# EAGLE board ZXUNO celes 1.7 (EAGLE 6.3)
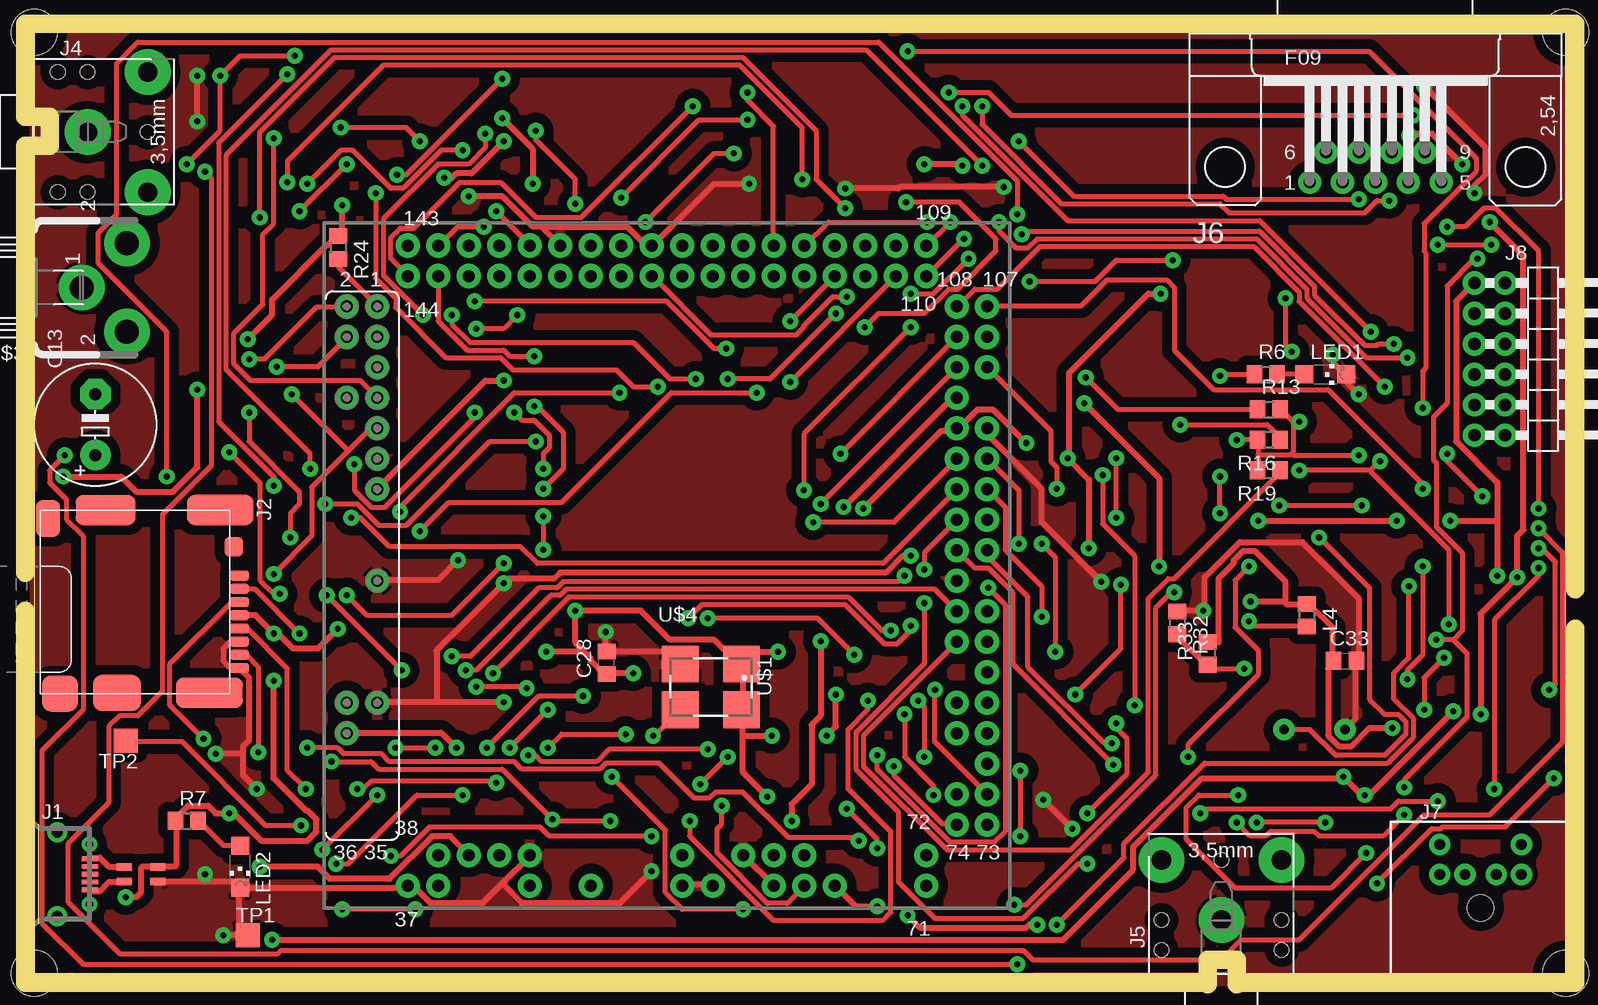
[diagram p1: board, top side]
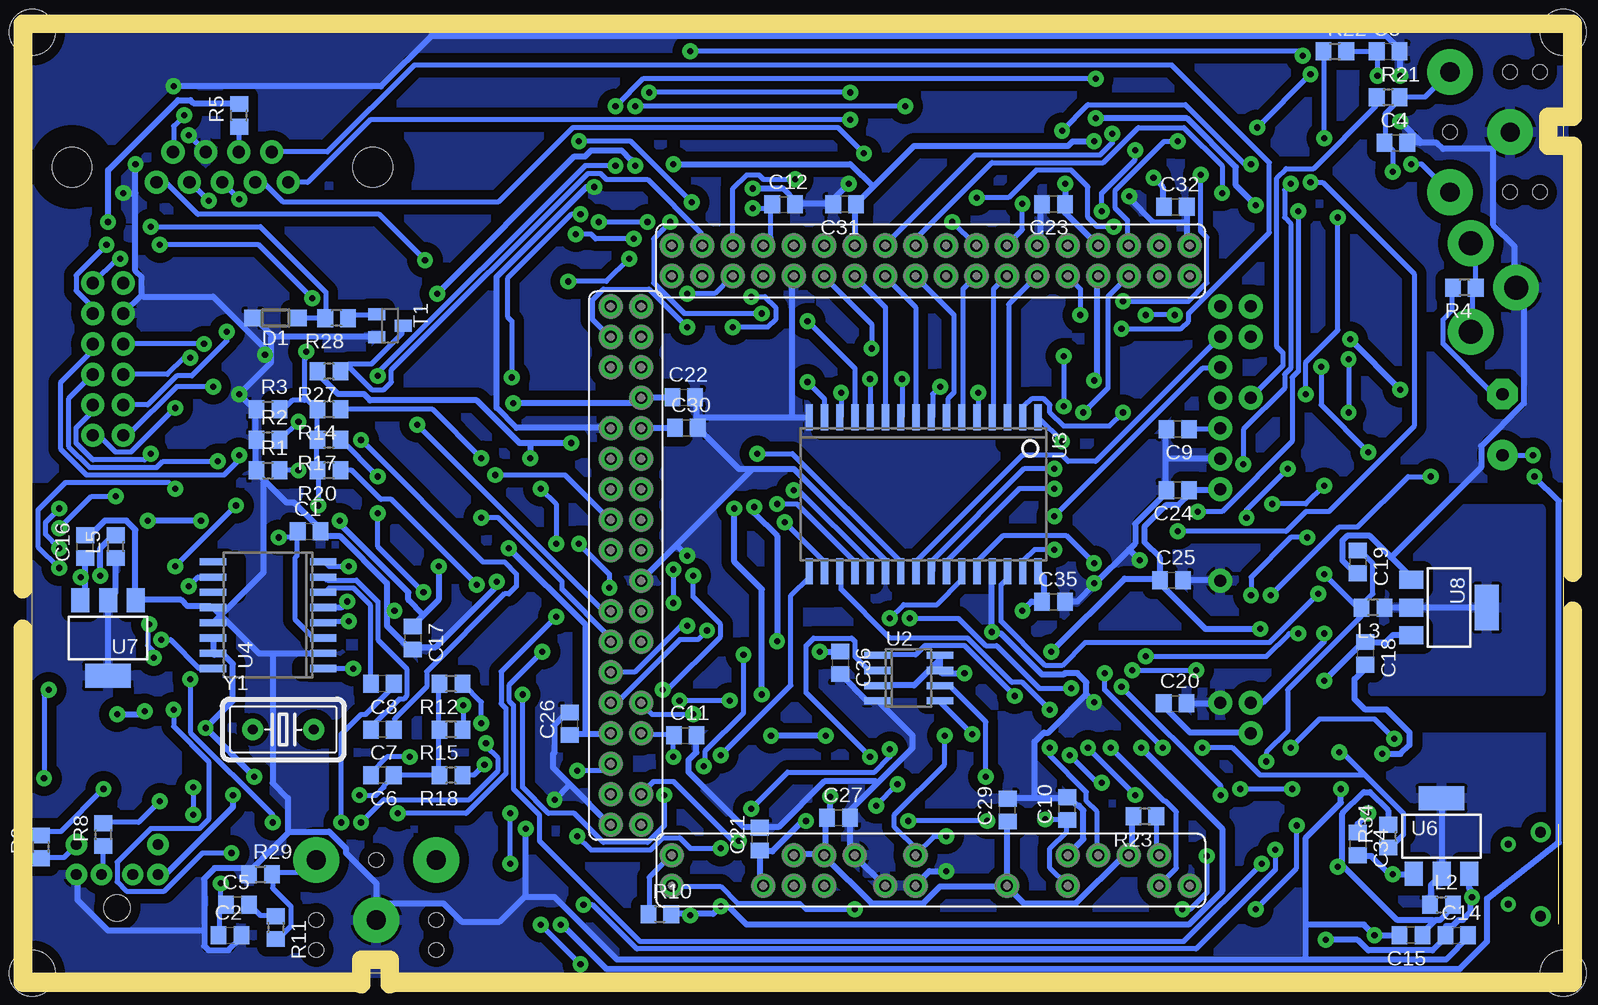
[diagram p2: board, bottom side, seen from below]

Size 127.61 x 78.41 mm. Coordinates in mm from the lower left corner, seen from the top.
Outline: 0,0 127.61,0 127.61,78.41 0,78.41 0,0
Copper layers (1*16): Top 0.035mm / dielectric 1.5mm / Bottom 0.035mm
Design rules "default *": minimum track width 16mil, minimum drill 20mil, track to track 8mil, track to pad 8mil, pad to pad 8mil, via to via 10mil, smd to smd 8mil, copper to edge 0mil, drill to drill 10mil, minimum pad ring 10mil, minimum via ring 16mil, stop-mask expansion 4mil, vias tented up to drill 0mil, thermal gap 10mil
Net classes: 0 default: width 0.381 mm, drill 0.203 mm, clearance 0.203 mm; 1 alimentacion: width 0.508 mm, drill 0.203 mm, clearance 0.203 mm
Holes 3.81 mm at 0,78.41 127.61,78.41 127.61,0 0,0
tRestrict: area 116.3,64.9 to 118.2,66.9; area 113.5,64.9 to 115.4,66.9; area 110.8,64.9 to 112.8,66.9; area 108,64.9 to 110,66.9; area 105.3,64.9 to 107.3,66.9; area 106.7,67.5 to 108.7,69.4; area 109.4,67.5 to 111.4,69.4; area 112.1,67.5 to 114,69.4; area 114.9,67.5 to 116.8,69.4; area 7.6,63.4 to 11.2,66.9; area 2.5,68.3 to 6.1,71.9; area 7.6,73.3 to 11.2,76.8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
bRestrict: area 108.7,19.8 to 109.7,20.8; area 103.6,19.8 to 104.7,20.9; area 61,31.3 to 63.4,32.2; area 43.6,31.6 to 46.6,32.3; area 43.6,44.1 to 46.5,45; area 110.6,31.6 to 111.3,34.4; area 113.8,33.9 to 114.7,34.5; area 104.5,25.1 to 105.2,25.7; area 104.5,29.6 to 105.4,34.5
vRestrict: area 50.8,21.4 to 58.4,27.8; area 102.2,24.1 to 113.7,35.6; area 92.7,-2.5 to 104.8,11.4; area 119.4,43.6 to 127,58.8; area -1.3,3.8 to 5.7,12.7; area 7,7.6 to 13.3,15.9; area 112.9,-0.3 to 128.1,12.4; area 96.3,64.3 to 102.6,78.9; area 121.3,64.3 to 127,78.9; area 99.6,74.7 to 124.3,78.5; area -2,64.4 to 11.9,76.5; area 0.6,20.3 to 18.4,40.6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
Milling: 15 lines

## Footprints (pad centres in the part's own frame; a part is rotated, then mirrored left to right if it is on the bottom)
C0805 = smd 1.3 x 1.5: 1 -0.95,0; 2 0.95,0
E5-10,5 = drill 1.016 pad 2.54: + -2.54,0 | drill 1.016 pad 2.54 octagon: - 2.54,0
SOD123 = smd 1.4 x 1.4: A 1.9,0; C -1.9,0
MICRO_USB = smd 1.35 x 0.4: 1 2.73,1.3; 2 2.73,0.65; 3 2.73,0; 4 2.73,-0.65; 5 2.73,-1.3 | drill 0.6 pad 1.27: P$1 2.7,2.5; P$2 2.7,-2.5 | drill 0.9 pad 1.676: P$3 0,3.5; P$4 0,-3.5
MICRO_SD_CONNECTOR = smd 0.8 x 1.6: 1 -2.03,8.2; 2 -0.93,8.2; 3 0.17,8.2; 4 1.27,8.2; 5 2.37,8.2; 6 3.47,8.2; 7 4.57,8.2; 8 5.67,8.2 | smd 2.54 x 5.588: 9 7.735,5.7; 14 -7.49,6.6 | smd 3 x 4: 10 7.735,-2 | smd 3 x 3: 11 7.81,-6.75 | smd 3 x 2: 12 -6.79,-7.75 | smd 2.5 x 5: 13 -7.49,-2.95 | smd 1.6 x 1.55: 15 -4.43,7.725
STX = drill 1.6 pad 3.81: P$1 -0.762,-0.127; P$2 4.242,-5.131; P$3 4.242,4.877 | hole 1.2: -3.251,4.877; -0.762,4.877; -0.762,-5.131; -3.251,-5.131; 4.242,-0.127
F09H = drill 1.016 pad 1.93: 1 -5.486,-1.27; 2 -2.743,-1.27; 3 0,-1.27; 4 2.743,-1.27; 5 5.486,-1.27; 6 -4.115,1.27; 7 -1.372,1.27; 8 1.372,1.27; 9 4.115,1.27 | hole 3.302: -12.522,0; 12.522,0
MDIN06SS = drill 0.9 pad 1.778: 1 1.3,8.5; 2 -1.3,8.5; 3 3.4,8.5; 4 -3.4,8.5; 5 3.4,11; 6 -3.4,11 | hole 2.2: 0,5.716
2X06/90 = drill 1.016 pad 1.93: 1 -6.35,-6.35; 2 -6.35,-3.81; 3 -3.81,-6.35; 4 -3.81,-3.81; 5 -1.27,-6.35; 6 -1.27,-3.81; 7 1.27,-6.35; 8 1.27,-3.81; 9 3.81,-6.35; 10 3.81,-3.81; 11 6.35,-6.35; 12 6.35,-3.81
CHOKE_COMM = smd 1.27 x 0.635: P$1 -1.4,0.6; P$2 -1.4,-0.6; P$3 1.4,-0.6; P$4 1.4,0.6
0805 = smd 1.3 x 1.5: 1 -0.95,0; 2 0.95,0
CHIPLED_1206 = smd 1.5 x 1.5: A 0,-1.75; C 0,1.75
R0805 = smd 1.3 x 1.5: 1 -0.95,0; 2 0.95,0
SOT23 = smd 1 x 1.4: 1 -0.95,-1.1; 2 0.95,-1.1; 3 0,1.1
TP20SQ = smd 2 x 2: TP 0,0
SO-08 = smd 0.6 x 2.2: 1 -1.905,-2.6; 2 -0.635,-2.6; 3 0.635,-2.6; 4 1.905,-2.6; 5 1.905,2.6; 6 0.635,2.6; 7 -0.635,2.6; 8 -1.905,2.6
SOIC32 = smd 0.6 x 2.2: 1 -9.525,-6.416; 2 -8.255,-6.416; 3 -6.985,-6.416; 4 -5.715,-6.416; 5 -4.445,-6.416; 6 -3.175,-6.416; 7 -1.905,-6.416; 8 -0.635,-6.416; 9 0.635,-6.416; 10 1.905,-6.416; 11 3.175,-6.416; 12 4.445,-6.416; 13 5.715,-6.416; 14 6.985,-6.416; 15 8.255,-6.416; 16 9.525,-6.416; 17 9.525,6.416; 18 8.255,6.416; 19 6.985,6.416; 20 5.715,6.416; 21 4.445,6.416; 22 3.175,6.416; 23 1.905,6.416; 24 0.635,6.416; 25 -0.635,6.416; 26 -1.905,6.416; 27 -3.175,6.416; 28 -4.445,6.416; 29 -5.715,6.416; 30 -6.985,6.416; 31 -8.255,6.416; 32 -9.525,6.416
SO16W = smd 0.6 x 2.2: 1 -4.445,-4.6; 2 -3.175,-4.6; 3 -1.905,-4.6; 4 -0.635,-4.6; 5 0.635,-4.6; 6 1.905,-4.6; 7 3.175,-4.6; 8 4.445,-4.6; 9 4.445,4.6; 10 3.175,4.6; 11 1.905,4.6; 12 0.635,4.6; 13 -0.635,4.6; 14 -1.905,4.6; 15 -3.175,4.6; 16 -4.445,4.6
SOT223 = smd 1.5 x 2: 1 -2.3,-3.15; 2 0,-3.15; 3 2.3,-3.15 | smd 3.8 x 2: 4 0,3.15
SM77H = smd 3.048 x 3.048: 1 -2.55,-1.9; 2 2.55,-1.9; 3 2.55,1.9; 4 -2.55,1.9
RCA_PACK = drill 2 pad 3.81: 1 0,-3.945; 2 3.688,-7.72; 2@1 -3.688,-7.72
TQ144_DIP_INCOMPLETO_2CARAS = drill 1 pad 2.007: P1 -24.13,21.59; P2 -26.67,21.59; P3 -24.13,19.05; P4 -26.67,19.05; P5 -24.13,16.51; P7 -24.13,13.97; P8 -26.67,13.97; P9 -24.13,11.43; P11 -24.13,8.89; P13 -24.13,6.35; P19 -24.13,-1.27; P27 -24.13,-11.43; P28 -26.67,-11.43; P30 -26.67,-13.97; P37 -21.59,-26.67; P39 -19.05,-26.67; P40 -19.05,-24.13; P42 -16.51,-24.13; P44 -13.97,-24.13; P45 -11.43,-26.67; P46 -11.43,-24.13; P49 -6.35,-26.67; P55 1.27,-26.67; P56 1.27,-24.13; P57 3.81,-26.67; P60 6.35,-24.13; P61 8.89,-26.67; P62 8.89,-24.13; P63 11.43,-26.67; P64 11.43,-24.13; P65 13.97,-26.67; P71 21.59,-26.67; P72 21.59,-24.13; P73 26.67,-21.59; P74 24.13,-21.59; P75 26.67,-19.05; P76 24.13,-19.05; P77 26.67,-16.51; P79 26.67,-13.97; P80 24.13,-13.97; P81 26.67,-11.43; P82 24.13,-11.43; P83 26.67,-8.89; P85 26.67,-6.35; P86 24.13,-6.35; P87 26.67,-3.81; P88 24.13,-3.81; P90 24.13,-1.27; P91 26.67,1.27; P92 24.13,1.27; P93 26.67,3.81; P94 24.13,3.81; P95 26.67,6.35; P96 24.13,6.35; P97 26.67,8.89; P98 24.13,8.89; P99 26.67,11.43; P100 24.13,11.43; P102 24.13,13.97; P103 26.67,16.51; P104 24.13,16.51; P105 26.67,19.05; P106 24.13,19.05; P107 26.67,21.59; P108 24.13,21.59; P109 21.59,26.67; P110 21.59,24.13; P111 19.05,26.67; P112 19.05,24.13; P113 16.51,26.67; P114 16.51,24.13; P115 13.97,26.67; P116 13.97,24.13; P117 11.43,26.67; P118 11.43,24.13; P119 8.89,26.67; P120 8.89,24.13; P121 6.35,26.67; P122 6.35,24.13; P123 3.81,26.67; P124 3.81,24.13; P125 1.27,26.67; P126 1.27,24.13; P127 -1.27,26.67; P128 -1.27,24.13; P129 -3.81,26.67; P130 -3.81,24.13; P131 -6.35,26.67; P132 -6.35,24.13; P133 -8.89,26.67; P134 -8.89,24.13; P135 -11.43,26.67; P136 -11.43,24.13; P137 -13.97,26.67; P138 -13.97,24.13; P139 -16.51,26.67; P140 -16.51,24.13; P141 -19.05,26.67; P142 -19.05,24.13; P143 -21.59,26.67; P144 -21.59,24.13
HC18U-V = drill 0.813 pad 1.778: 1 -2.54,0; 2 2.54,0

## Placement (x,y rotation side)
C1  15pF  [C0805]  104.52,36.83 0 bottom
C2  10nF  [C0805]  111.12,3.17 0 bottom
C3  10nF  [C0805]  14.61,76.83 0 bottom
C4  10nF  [C0805]  13.97,69.22 0 bottom
C5  100nF  [C0805]  110.49,5.71 0 bottom
C6  100nF  [C0805]  98.42,16.51 180 bottom
C7  100nF  [C0805]  98.42,20.32 180 bottom
C8  100nF  [C0805]  98.42,24.13 180 bottom
C9  100nF  [C0805]  32.14,45.35 180 bottom
C10  100nF  [C0805]  41.34,13.73 90 bottom
C11  100nF  [C0805]  73.18,19.82 0 bottom
C12  100nF  [C0805]  64.98,64.07 0 bottom
C13  220uF  [E5-10,5]  5.08,45.72 90 top
C14  4,7uF  [C0805]  8.89,3.17 0 bottom
C15  4,7uF  [C0805]  12.7,3.17 180 bottom
C16  4,7uF  [C0805]  123.19,35.56 90 bottom
C17  4,7uF  [C0805]  95.89,27.94 270 bottom
C18  4,7uF  [C0805]  16.51,26.67 270 bottom
C19  4,7uF  [C0805]  17.14,34.29 270 bottom
C20  100nF  [C0805]  32.36,22.49 0 bottom
C21  100nF  [C0805]  66.96,11.19 90 bottom
C22  100nF  [C0805]  73.31,48.02 0 bottom
C23  100nF  [C0805]  42.5,64.09 180 bottom
C24  100nF  [C0805]  32.14,40.27 180 bottom
C25  100nF  [C0805]  32.67,32.78 0 bottom
C26  100nF  [C0805]  82.79,20.8 90 bottom
C27  100nF  [C0805]  60.41,12.98 0 bottom
C28  100nF  [C0805]  47.69,25.88 90 top
C29  100nF  [C0805]  46.33,13.6 90 bottom
C30  100nF  [C0805]  73.09,45.48 0 bottom
C31  100nF  [C0805]  59.9,64.09 180 bottom
C32  100nF  [C0805]  32.34,63.87 0 bottom
C33  100nF  [C0805]  109.22,26.04 0 top
C34  4,7uF  [C0805]  17.14,10.79 270 bottom
C35  100nF  [C0805]  42.5,30.96 0 bottom
C36  100nF  [C0805]  60.28,25.88 270 bottom
D1  [SOD123]  107.31,54.61 180 bottom
J1  CON_MICRO_USB  [MICRO_USB]  1.91,8.26 0 top
J2  MICROSD_SPI_MODE  [MICRO_SD_CONNECTOR]  8.89,31.11 270 top
J4  JACK_STEREO  [STX]  5.21,70.23 0 top
J5  JACK_STEREO  [STX]  98.81,5.21 90 top
J6  [F09H]  111.76,67.18 0 top
J7  [MDIN06SS]  120.52,-0.25 0 top
J8  JTAG_RGB  [2X06/90]  126.36,51.18 270 top
L1  BOBINA_VCC_ZXUNO  [CHOKE_COMM]  8.89,8.26 0 top
L2  FERRITE  [0805]  10.16,5.71 0 bottom
L3  FERRITE  [0805]  15.88,30.48 180 bottom
L4  FERRITE  [0805]  106.05,29.84 270 top
L5  FERRITE  [0805]  120.65,35.56 90 bottom
LED1  [CHIPLED_1206]  107.57,49.91 270 top
LED2  [CHIPLED_1206]  17.14,8.89 180 top
R1  75  [R0805]  107.95,41.91 0 bottom
R2  75  [R0805]  107.95,44.45 0 bottom
R3  75  [R0805]  107.95,46.99 0 bottom
R4  75  [R0805]  8.26,57.15 180 bottom
R5  270  [R0805]  110.36,71.5 90 bottom
R6  220  [R0805]  102.62,49.91 0 top
R7  220  [R0805]  12.7,12.7 0 top
R8  270  [R0805]  121.67,11.56 90 bottom
R9  270  [R0805]  126.87,10.54 90 bottom
R10  330  [R0805]  75.3,4.94 0 bottom
R11  470  [R0805]  107.31,3.81 270 bottom
R12  470  [R0805]  92.71,24.13 180 bottom
R13  470  [R0805]  102.87,46.99 0 top
R14  470  [R0805]  102.87,46.99 180 bottom
R15  1K  [R0805]  92.71,20.32 180 bottom
R16  1K  [R0805]  102.87,44.45 180 top
R17  1K  [R0805]  102.87,44.45 180 bottom
R18  2K  [R0805]  92.71,16.51 180 bottom
R19  2K  [R0805]  102.87,41.91 180 top
R20  2K  [R0805]  102.87,41.91 180 bottom
R21  3K9  [R0805]  14.61,73.03 0 bottom
R22  3K9  [R0805]  19.05,76.83 0 bottom
R23  4K7  [R0805]  34.88,13.07 180 bottom
R24  4K7  [R0805]  25.32,60.48 270 top
R27  1OK  [R0805]  102.87,50.16 180 bottom
R28  10K  [R0805]  102.23,54.61 180 bottom
R29  10K  [R0805]  108.58,8.26 0 bottom
R32  0  [R0805]  95.25,29.21 270 top
R33  0  [R0805]  97.79,26.67 90 top
R34  10K  [R0805]  14.61,11.43 90 bottom
T1  BC846  [SOT23]  97.79,53.98 270 bottom
TP1  TPTP20SQ  [TP20SQ]  17.78,3.17 0 top
TP2  TPTP20SQ  [TP20SQ]  7.64,19.38 180 top
U2  W25X40BV  [SO-08]  54.56,24.61 270 bottom
U3  CY62148EV30  [SOIC32]  53.32,39.93 180 bottom
U4  AD724JR  [SO16W]  107.95,29.84 90 bottom
U6  LD117AS33TR  [SOT223]  10.16,11.43 0 bottom
U7  LD117AS25TR  [SOT223]  121.28,27.94 180 bottom
U8  LD117AS12TR  [SOT223]  9.53,30.48 270 bottom
U$1  SIT1602AC-83  [SM77H]  56.38,23.87 180 top
U$3  RCA_VIDEO  [RCA_PACK]  0,57.15 90 top
U$4  [TQ144_DIP_INCOMPLETO_2CARAS]  52.72,33.98 0 top
Y1  4.43M/3.58M  [HC18U-V]  106.68,20.32 0 bottom

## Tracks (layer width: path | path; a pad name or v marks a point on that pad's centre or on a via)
1.2V  (via drill 0.51)
  Top 0.406: v24.77,17.65 28.07,17.65 28.7,17.02 38.99,17.02 v43.18,12.83 43.31,12.7 v48.01,12.7 | v19.94,33.27 23.11,36.45 23.11,40.51 26.16,43.56 | 26.16,43.56 27.94,45.34 28.57,45.34 U$4.P9 | v67.56,63.75 65.15,66.17 65.15,70.23 59.05,76.33 25.02,76.33 18.8,70.1 v18.8,62.99 | 26.16,43.56 v21.46,48.26 | v74.17,18.03 74.17,22.23 v73.66,22.73 | v69.47,22.73 69.47,21.97 67.82,20.32 67.82,15.37 71.37,11.81 71.37,5.08 70.74,4.45 61.59,4.45 54.61,11.43 v54.61,12.7
  Bottom 0.406: C9.1 31.11,45.34 28.7,45.34 U$4.P9 | U$4.P45 41.4,7.37 42.8,8.76 42.8,10.41 41.4,11.81 41.4,12.7 C10.1 41.53,12.83 v43.18,12.83 | v24.77,17.65 24.77,18.41 22.99,20.19 22.99,23.62 16.89,29.72 16.89,30.35 L3.2 | U$4.P115 66.67,60.71 66.04,61.34 66.04,64.01 C12.1 66.17,63.75 v67.56,63.75 | C19.1 17.14,35.18 16.89,35.18 15.88,34.16 15.88,31.62 16.89,30.61 L3.2 | v19.94,33.27 17.4,30.73 17.02,30.73 L3.2 | v18.8,62.99 18.8,53.59 21.46,50.93 v21.46,48.26 | U$4.P80 76.83,19.94 74.17,19.94 C11.1 74.17,19.68 v74.17,18.03 | v69.47,22.73 v73.66,22.73 | v48.01,12.7 v54.61,12.7
2.5V  (via drill 0.51)
  Top 0.508: v63.12,12.7 63.12,14.1 64.77,15.75 64.77,20.7 65.53,21.46 v65.53,27.69 | v67.44,38.86 76.45,47.88 76.83,47.88 U$4.P102 | v41.53,65.79 41.53,68.71 v38.99,71.25 | v25.65,64.01 25.65,61.85 25.4,61.59 R24.1 25.15,61.34 24.51,60.71 24.38,60.71 19.81,56.13 19.81,54.86 v17.78,52.83 | v70.23,5.59 68.45,5.59 66.8,7.24 U$4.P65 | v35.18,18.8 33.91,20.07 26.16,20.07 U$4.P30 | 121.92,37.72 121.92,40.89 118.49,44.32 118.49,56.01 J8.1 | 121.92,37.72 v121.92,33.15 | v93.73,33.91 93.73,41.27 v87.5,47.5 | v13.59,48.64 13.59,42.16 11.56,40.13 8.51,40.13 7.24,41.4 v2.41,41.4 | v83.57,4.06 82.93,4.06 82.68,3.81 73.79,3.81 v72.77,4.83 | v117.98,37.72 121.92,37.72 | v101.98,37.72 v113.54,37.72
  Bottom 0.508: C22.1 74.3,48.01 76.83,48.01 U$4.P102 77.09,47.88 77.47,47.5 v87.5,47.5 | U$4.P137 38.86,60.71 41.53,63.37 41.53,64.01 C23.1 41.53,64.26 v41.53,65.79 | U$4.P65 66.8,7.37 66.93,7.49 66.93,10.16 C21.1 66.67,10.16 65.91,10.16 63.37,12.7 v63.12,12.7 | C20.1 33.27,22.48 33.27,22.23 31.11,20.07 26.16,20.07 U$4.P30 | v65.53,27.69 65.53,36.45 67.44,38.35 v67.44,38.86 | v38.99,71.25 31.37,71.25 27.3,67.18 27.3,65.66 v25.65,64.01 | 72.77,4.95 70.87,4.95 v70.23,5.59 70.1,5.46 69.47,5.46 68.07,4.06 31.24,4.06 28.45,6.86 28.45,12.06 v35.18,18.8 | 72.77,4.95 74.3,4.95 R10.2 | v121.92,33.15 121.92,35.43 120.9,36.45 120.65,36.45 L5.2 | 95,29.84 93.73,31.11 v93.73,33.91 | 95,29.84 95.89,28.96 C17.1 | v13.59,48.64 v17.78,52.83 | v2.41,41.4 0.38,39.37 0.38,10.92 6.35,6.22 6.35,2.67 8.64,0.38 79.76,0.38 83.44,4.06 v83.57,4.06 | v72.77,4.83 72.77,4.95 | v113.54,37.72 v117.98,37.72 | v101.98,37.72 101.98,37.47 96.27,31.75 96.27,31.11 95,29.84
3.3V  (via drill 0.51)
  Top 0.508: v49.91,25.02 47.75,25.02 C28.1 47.5,24.89 46.35,26.04 46.35,26.29 45.72,26.92 | 45.72,26.92 45.09,27.56 v45.09,30.23 50.55,30.23 52.96,27.81 56.64,27.81 58.67,25.78 U$1.1 | U$1.1 59.05,25.53 59.05,21.97 U$1.4 59.05,21.72 59.05,19.81 | 59.05,19.81 59.05,16.76 v61.09,14.73 | v42.67,26.8 45.59,26.8 45.72,26.92 | J2.4 18.41,29.84 v19.94,28.32 20.07,28.19 20.45,28.19 21.59,27.05 23.62,27.05 v25.27,28.7 | v61.98,26.8 57.91,26.8 U$1.1 | v69.09,38.73 75.56,45.21 76.71,45.21 U$4.P100 77.09,45.47 78.61,46.99 79.88,46.99 v82.68,44.2 | v66.8,23.24 66.8,20.57 v66.04,19.81 | 59.05,19.81 v61.47,19.81 | v39.12,49.4 37.59,49.4 28.57,40.39 U$4.P13 | v18.8,8.89 23.62,8.89 24.64,7.87 29.59,7.87 33.15,11.43 34.67,11.43 36.2,9.91 U$4.P42 | v34.16,66.29 34.8,66.29 35.18,66.67 36.45,66.67 v39.12,69.34 | v87.88,35.43 87.88,41.15 v86.11,42.93 86.23,43.05 86.23,50.04 92.84,56.64 v93.85,56.64 | v74.17,67.44 77.22,67.44 v77.34,67.31
  Bottom 0.508: U$4.P13 28.7,40.26 31.11,40.26 C24.1 31.11,40.01 32.13,38.99 33.15,38.99 34.92,37.21 34.92,35.94 33.66,34.67 33.66,32.89 C25.1 | C30.1 74.04,45.47 76.83,45.47 U$4.P100 | U$4.P121 59.05,60.71 59.05,63.88 C31.1 58.8,64.26 57.53,65.53 | U3.32 43.69,33.4 43.31,33.02 43.31,31.37 43.43,31.24 43.43,30.99 C35.1 43.69,30.99 44.32,30.99 v45.09,30.23 | v49.91,25.02 51.82,25.02 51.94,25.15 U2.7 51.94,25.4 51.94,26.04 | 51.94,26.04 51.94,26.42 U2.8 | U2.3 57.15,24 54.1,24 52.07,26.04 51.94,26.04 | R23.2 35.94,12.95 35.94,10.16 36.2,9.91 U$4.P42 36.45,9.78 36.7,9.78 40.64,5.84 44.96,5.84 46.23,7.11 U$4.P49 | C29.1 46.35,12.57 46.35,7.37 U$4.P49 | U$4.P62 61.59,9.91 61.47,10.03 61.47,12.95 C27.1 61.34,13.21 61.09,13.46 v61.09,14.73 | U$4.P49 46.61,7.24 51.94,7.24 53.34,5.84 57.66,5.84 61.47,9.65 U$4.P62 | U$4.P64 64.14,9.91 61.85,9.91 U$4.P62 | v42.67,26.8 36.58,32.89 33.91,32.89 C25.1 | v19.94,28.32 19.94,27.69 25.02,22.61 26.04,22.61 U$4.P28 | v61.98,26.8 60.33,26.8 C36.1 | v69.09,38.73 69.09,34.29 66.8,32 v66.8,23.24 | v61.47,19.81 v66.04,19.81 | 10.79,4.32 10.67,4.45 10.29,4.45 9.27,5.46 9.27,5.71 L2.2 | 10.79,4.32 11.68,3.43 11.68,3.17 C15.1 | R34.2 14.61,13.59 16.13,15.11 16.64,15.11 18.41,13.34 18.41,9.02 | 18.41,9.02 13.84,4.45 10.92,4.45 10.79,4.32 | v39.12,49.4 38.86,49.66 38.86,58.04 U$4.P138 | v18.8,8.89 18.54,8.89 18.41,9.02 | v25.27,28.7 29.84,28.7 33.66,32.51 C25.1 | v34.16,66.29 33.4,65.53 33.4,63.88 C32.1 | v39.12,69.34 40.89,69.34 41.27,68.96 54.1,68.96 57.53,65.53 | 81.53,19.94 79.5,19.94 U$4.P79 | 81.53,19.94 82.68,19.94 C26.1 | v82.68,44.2 86.11,44.2 | 86.11,44.2 87,44.2 90.55,47.75 99.44,47.75 99.95,48.26 102.11,48.26 103.76,49.91 103.76,50.16 R27.2
  Bottom 0.508: 81.53,19.94 81.53,29.08 v87.88,35.43 | 86.11,44.2 v86.11,42.93 | 57.53,65.53 59.44,67.44 v74.17,67.44 | v77.34,67.31 77.72,67.69 77.72,67.82 78.49,68.58 81.03,68.58 81.53,68.07 82.42,68.07 v93.85,56.64
5V  (via drill 0.51)
  Top 0.508: v7.62,6.35 8.51,6.35 8.89,6.73 8.89,8.76 9.02,8.89 10.03,8.89 L1.P$4 10.41,8.89 11.68,8.89 11.81,9.02 11.81,12.7 R7.1 11.68,12.83 12.83,13.97 14.48,13.97 15.11,13.34 v16.26,13.34 16.38,13.21 16.76,13.21 18.92,11.05 22.73,11.05 23.5,11.81 23.5,12.83 22.73,13.59 22.61,13.59 19.94,16.26 v19.94,24.38 | 104.27,30.99 104.27,30.86 104.39,30.73 106.05,30.73 L4.1 106.17,30.61 106.43,30.61 108.2,28.83 108.2,26.29 C33.1 108.2,25.78 107.82,25.4 107.82,19.81 108.71,18.92 109.73,18.92 111.25,20.45 v113.16,20.45 | 104.27,30.99 104.27,32.64 101.73,35.18 100.71,35.18 99.95,34.42 99.95,34.16 98.68,32.89 98.68,27.56 97.79,27.56 R33.2 | 104.27,30.99 v101.35,30.99 | v121.28,62.61 124.08,59.82 124.08,36.96 123.57,36.45 v123.57,33.02 120.52,29.97 v120.52,21.59 | v118.24,21.84 111.38,14.99 111,14.99 v110.87,14.86 110.62,14.86 v109.09,16.38 108.97,16.26 97.28,16.26 91.57,10.54 91.57,8.64 85.72,2.79 v19.81,2.79
  Bottom 0.508: 7.75,6.35 7.75,6.99 7.87,7.11 7.87,8.26 U6.3 | 7.75,6.35 7.75,5.08 8.38,4.45 8.76,4.45 9.27,3.94 9.78,3.94 9.78,3.17 C14.1 9.78,3.05 10.92,1.91 16.26,1.91 17.14,2.79 v19.81,2.79 | 14.86,27.56 16.51,27.56 C18.1 16.64,27.43 16.89,27.43 v19.94,24.38 | 14.86,27.56 14.22,28.19 12.7,28.19 U8.3 | 14.73,27.43 14.86,27.56 | v7.62,6.35 7.75,6.35 | U4.5 101.85,30.48 v101.35,30.99 | 123.19,33.02 123.19,31.5 123.57,31.11 U7.3 | 123.19,33.02 C16.1 | v121.28,62.61 121.28,66.93 115.44,72.77 114.43,72.77 114.17,72.52 110.36,72.52 R5.2 | 123.19,33.02 v123.57,33.02 | C34.1 17.14,12.45 v16.26,13.34 | U4.14 112.52,27.94 112.52,26.67 U4.15 112.39,26.54 111.63,26.54 110.87,25.78 110.87,22.73 v113.16,20.45 v109.09,16.38 | v110.87,14.86 110.87,13.84 116.46,8.26 117.09,8.26 J7.4 | v118.24,21.84 118.49,21.59 v120.52,21.59
B  (via drill 0.51)
  Top 0.406: 111.38,41.91 v105.41,41.91 | v112.14,42.67 111.38,41.91 | v100.33,14.86 97.03,14.86 96.01,13.84 96.01,11.18 100.08,7.11 108.08,7.11 v111,10.03 | v115.82,21.97 115.82,24.64 v117.47,26.29 | v117.86,29.08 117.86,35.31 111.38,41.78 111.38,41.91
  Bottom 0.406: R12.2 93.73,24.13 93.73,20.45 R15.2 93.73,20.19 93.73,16.64 R18.2 C6.1 97.54,16.38 98.3,15.62 98.3,15.49 98.93,14.86 v100.33,14.86 | v105.41,41.91 R1.2 | v112.14,42.67 116.71,42.67 117.22,42.16 122.81,42.16 124.59,43.94 124.59,47.88 J8.8 | v111,10.03 113.41,10.03 116.59,6.86 119.76,6.86 120.52,7.62 120.52,9.27 117.73,12.06 113.67,12.06 112.9,12.83 112.9,17.65 115.82,20.57 v115.82,21.97 | v117.47,26.29 117.35,26.42 117.35,26.67 117.98,27.3 117.98,28.96 v117.86,29.08
B0  (via drill 0.51)
  Top 0.406: v89.92,17.4 81.53,25.78 81.53,31.75 79.5,33.78 78.36,33.78 76.96,35.18 U$4.P92
  Bottom 0.406: R18.1 90.81,16.51 v89.92,17.4
B1  (via drill 0.51)
  Top 0.406: v91.69,22.35 91.69,34.8 89.03,37.47 v89.03,41.53
  Bottom 0.406: v91.69,22.35 91.69,20.32 R15.1 | v89.03,41.53 83.19,41.53 79.5,37.85 U$4.P93
B2  (via drill 0.51)
  Top 0.406: v90.17,20.83 90.17,20.45 91.06,19.56 91.06,16.64 v87.76,13.34 | v87.76,9.14 87,9.14 82.42,4.57 75.06,4.57 72.01,7.62 72.01,13.46 68.45,17.02 68.45,20.07 74.17,25.78 v74.17,30.86 | v74.17,33.66 74.17,35.05 76.83,37.72 U$4.P94
  Bottom 0.406: v90.17,20.83 90.17,22.61 91.69,24.13 R12.1 | v87.76,9.14 v87.76,13.34 | v74.17,33.66 v74.17,30.86
CLK  (via drill 0.51)
  Top 0.406: v22.23,12.32 19.3,12.32 12.32,19.3 7.75,19.3 TP2.TP | v31.75,5.33 v25.65,5.33 | v29.72,9.78 30.48,9.78 32.89,12.19 42.16,12.19 42.93,11.43 v51.44,11.43 | v51.56,19.81 51.69,19.81 53.72,21.84 U$1.3
  Bottom 0.406: v22.23,12.32 22.23,8.76 v25.65,5.33 | v31.75,5.33 31.11,5.33 29.72,6.73 v29.72,9.78 | v51.44,11.43 52.45,11.43 53.98,9.91 U$4.P56 53.85,10.29 55.75,12.19 55.75,13.21 51.56,17.4 v51.56,19.81
CSYNC  (via drill 0.51)
  Top 0.406: 118.24,27.81 v116.84,27.81 | 118.24,27.81 119,28.57 119,35.05 116.84,37.21 116.84,42.55 116.59,42.8 116.59,46.35 117.73,47.5 117.73,57.28 120.02,59.56 v120.27,59.56 | v89.79,19.18 89.15,19.18 82.8,25.53 82.8,31.37 79.5,34.67 79.5,35.18 U$4.P91 | v100.2,12.57 101.35,11.43 102.62,11.43 103,11.81 106.68,11.81 107.06,11.43 112.39,11.43 v114.17,13.21 | v114.17,15.49 114.17,16.13 119.38,21.34 119.38,26.67 118.24,27.81
  Bottom 0.406: U4.16 113.67,25.4 116.08,27.81 v116.84,27.81 | v120.27,59.56 120.52,59.56 J8.2 | v89.79,19.18 89.79,18.92 88.77,17.91 88.77,16.89 91.19,14.48 98.3,14.48 v100.2,12.57 | v114.17,15.49 v114.17,13.21
EAR
  Bottom 0.406: 101.35,50.67 101.85,50.16 R27.1 | 101.35,50.67 101.22,50.8 99.31,50.8 96.77,53.34 96.77,53.98 T1.3 | 101.35,50.67 99.31,48.64 98.3,48.64 97.66,49.28 97.66,50.29 81.28,66.67 80.26,66.67 79.76,66.17 76.33,66.17 71.88,61.72 71.88,60.71 U$4.P111
FLASH_CS  (via drill 0.51)
  Top 0.406: v45.72,23.11 42.04,23.11 v37.72,18.8
  Bottom 0.406: v45.72,23.11 49.91,27.3 53.21,27.3 53.98,26.54 57.15,26.54 U2.1 | v37.72,18.8 33.27,14.35 33.15,14.35 32.26,13.46 32.26,8.76 33.66,7.37 U$4.P39
FLASH_MISO  (via drill 0.51)
  Top 0.406: v55.5,15.75 v57.78,18.03 | v57.28,13.97 57.28,12.45 56.9,12.06 56.9,10.03 61.09,5.84 62.74,5.84 64.14,7.24 U$4.P63
  Bottom 0.406: v57.78,18.03 63.12,23.37 63.12,27.3 62.48,27.94 59.31,27.94 59.05,27.69 59.05,26.42 57.91,25.27 57.28,25.27 U2.2 | v57.28,13.97 v55.5,15.75
FLASH_MOSI  (via drill 0.51)
  Top 0.406: v49.28,19.94 43.94,19.94 v42.8,18.8
  Bottom 0.406: v49.28,19.94 51.94,22.61 U2.5 | v42.8,18.8 42.8,18.16 39.75,15.11 39.75,14.35 38.86,13.46 38.86,9.91 U$4.P44
FLASH_SCK  (via drill 0.51)
  Top 0.406: 74.3,7.24 U$4.P71 | v48.13,16.38 52.58,11.94 52.58,6.73 53.98,5.33 v59.05,5.33
  Bottom 0.406: v48.13,16.38 48.13,20.95 51.05,23.88 51.94,23.88 U2.6 | v59.05,5.33 63.12,5.33 63.63,5.84 68.83,5.84 70.23,7.24 74.3,7.24 U$4.P71
G  (via drill 0.51)
  Top 0.406: v100.2,44.45 R16.2 101.98,44.32 101.98,43.18 | 101.98,43.18 101.98,41.91 R19.2 | R13.2 103.89,46.99 104.9,45.97 v105.41,45.97 104.9,45.85 104.9,43.43 104.78,43.31 | 101.98,43.18 104.65,43.18 104.78,43.31 | v110.36,43.18 104.9,43.18 104.78,43.31
  Bottom 0.406: v100.2,44.45 90.04,34.29 88.27,34.29 87.25,33.27 87.25,32.26 87.88,31.62 88.27,31.62 94.74,25.15 94.74,23.88 97.41,21.21 97.41,20.32 C7.1 | 122.56,52.96 J8.6 122.68,52.32 122.68,51.82 125.22,49.28 125.22,43.69 123.06,41.53 111.63,41.53 110.36,42.8 v110.36,43.18 | v105.41,45.97 106.93,44.45 R2.2
G0
  Top 0.406: R19.1 103.76,41.91 103.76,41.66 95,32.89 94.49,32.89 92.84,31.24 92.84,16.76 86.36,10.29 76.07,10.29 69.09,17.27 69.09,19.81 76.83,27.56 U$4.P86
G1  (via drill 0.51)
  Top 0.406: v95.5,45.72 102.74,45.72 103.76,44.7 103.76,44.45 R16.1
  Bottom 0.406: v95.5,45.72 80.01,30.23 79.5,30.23 U$4.P87
G2  (via drill 0.51)
  Top 0.406: R13.1 90.3,46.99 v87.63,49.66 | v81.92,63.25 81.92,66.04 70.36,77.6 8.64,77.6 6.86,75.82 6.86,63.25 5.33,61.72 5.33,59.18 11.05,53.47 v11.05,41.4 | v30.61,25.27 v24.38,31.5 | v35.94,25.27 36.83,25.27 43.05,31.5 43.81,31.5 44.32,32 75.06,32 76.83,30.23 U$4.P88
  Bottom 0.406: v87.63,49.66 87.63,54.36 88.01,54.74 88.01,57.91 82.68,63.25 v81.92,63.25 | v11.05,41.4 12.95,41.4 17.14,37.21 18.67,37.21 v24.38,31.5 | v35.94,25.27 v30.61,25.27
GND  (via drill 0.51)
  Top 0.508: v13.59,70.99 v13.59,74.8 | U$4.P55 54.1,7.37 56.52,7.37 U$4.P57 | 53.85,25.78 U$1.2 53.59,25.78 52.58,26.8 47.75,26.8 C28.2 47.62,27.05 v47.62,28.45 | U$4.P61 61.59,7.37 59.18,9.78 U$4.P60 | v15.75,3.17 TP1.TP 17.02,3.3 17.02,6.99 LED2.C | 14.22,7.62 16.76,7.62 17.14,7.24 LED2.C | 14.22,7.62 10.41,7.62 L1.P$3 | 14.22,7.62 v14.22,8.26 | 38.99,7.49 41.27,9.78 U$4.P46 | 38.99,7.49 37.34,5.84 33.02,5.84 31.62,7.24 31.37,7.24 U$4.P37 30.99,7.11 17.4,7.11 LED2.C | v59.56,65.79 56.64,65.79 51.56,60.71 U$4.P127 51.31,60.83 50.8,60.83 49.4,62.23 42.55,62.23 42.42,62.1 | v36.2,64.77 38.99,64.77 41.53,62.23 42.29,62.23 42.42,62.1 | 42.42,62.1 43.81,60.71 U$4.P133 | v110.36,48.26 109.47,49.15 109.47,49.78 LED1.C 109.22,49.91 108.2,50.93 v108.2,51.56 | 38.99,7.49 40.64,5.84 48.77,5.84 v51.44,8.51 | Y1.1 110.11,21.21 110.11,26.04 C33.2 110.36,26.16 110.36,31.24 105.66,35.94 100.46,35.94 97.54,33.02 97.54,30.35 v97.41,30.23 95.25,30.23 R32.1 | v35.31,34.42 33.66,32.77 28.83,32.77 U$4.P19 | J2.6 17.02,27.56 16.26,27.56 15.75,27.05 15.75,26.04 16.26,25.53 17.02,25.53 J2.8 17.27,25.27 17.91,24.64 17.91,19.43 17.4,18.92 17.4,18.29 | v39.12,22.61 33.53,22.61 | 33.53,22.61 28.83,22.61 U$4.P27 | v86.49,12.06 v84.07,14.48 | 33.53,22.61 33.53,26.92 v39.12,32.51 39.5,32.89 43.31,32.89 43.81,33.4 70.99,33.4 72.39,34.8 v73.03,34.8 | 17.4,18.29 17.4,16.51 v18.54,15.37 | v88.9,32.64 83.95,37.59 83.95,40.39 79.5,44.83 79.5,45.34 U$4.P99 | v67.56,65.41 72.01,65.41 72.14,65.53 v80.77,65.53 | v114.55,69.85 115.19,69.85 115.32,69.98 116.46,69.98 v119,67.44 | v120.02,65.02 120.02,65.66 120.9,66.55 120.9,68.83 v115.82,73.91
  Top 0.508: 17.4,18.29 v15.11,18.29
  Bottom 0.508: 11.94,69.22 10.54,69.22 10.03,68.71 5.84,68.71 | 11.94,69.22 C4.2 | J4.P$1 5.84,68.71 | v13.59,74.8 13.59,76.83 C3.2 13.59,76.96 14.73,78.11 94.36,78.11 98.55,73.91 v115.82,73.91 | v13.59,70.99 11.94,69.34 11.94,69.22 | 5.84,68.71 5.84,62.36 4.06,60.58 4.06,57.28 U$3.1 3.94,56.9 3.3,56.26 3.3,47.5 6.86,43.94 6.86,42.16 14.35,34.67 | 33.15,42.93 33.15,40.51 C24.2 33.15,40.01 35.69,37.47 35.69,35.81 36.2,35.31 | 33.15,42.93 33.15,45.34 C9.2 | 33.15,42.93 28.7,42.93 U$4.P11 | C25.2 31.62,32.77 28.7,32.77 U$4.P19 | C20.2 31.37,22.48 28.7,22.48 U$4.P27 | 72.26,46.35 72.26,48.01 C22.2 | 72.26,46.35 72.26,45.59 C30.2 72.01,45.34 68.71,42.04 67.69,42.04 | 67.69,42.04 64.14,42.04 56.52,34.42 56.52,33.53 U3.22 | 72.26,46.35 64.26,46.35 | 64.26,46.35 62.87,46.35 U3.16 | 73.91,35.69 67.69,41.91 67.69,42.04 | 73.91,35.69 76.83,32.77 U$4.P90 | 64.26,46.35 64.26,58.04 U$4.P118 | U$4.P57 56.64,7.37 58.93,9.65 U$4.P60 59.18,9.91 59.44,10.16 59.44,12.95 C27.2 59.44,13.59 57.15,15.88 | C15.2 v15.75,3.17 16.64,4.06 21.46,4.06 | U6.1 12.57,8.26 v14.22,8.26 14.35,8.13 16,9.78 17.14,9.78 C34.2 | 57.15,22.73 U2.4 | U$4.P46 41.27,9.91 40.01,11.18 40.01,13.59 40.39,13.97 40.51,13.97 41.15,14.61 C10.2 41.53,14.61 44.07,14.61 | v59.56,65.79 60.96,64.39 C31.2 60.96,64.14 64.01,64.14 C12.2 64.01,64.39 65.02,65.41 v67.56,65.41 | 31.37,62.61 31.37,60.83 31.24,60.71 U$4.P143 | 31.37,62.61 31.37,63.75 C32.2 | C23.2 43.56,64.01 43.56,60.96 43.81,60.71 U$4.P133 | 31.37,62.61 34.16,62.61 36.2,64.64 v36.2,64.77 | 107.57,26.67 108.71,26.67 111.89,29.84 | 107.57,26.67 U4.2 | 111.89,29.84 112.52,30.48 U4.12 112.78,30.61 114.68,30.61 115.19,31.11 118.75,31.11 U7.1 119,31.11 119,36.96 119.76,37.72 121.54,37.72 122.68,36.58 123.19,36.58 C16.2
  Bottom 0.508: 111.89,29.84 112.52,29.21 U4.13 | 108.2,41.02 108.84,41.66 108.84,41.91 R1.1 108.97,42.04 108.97,44.45 R2.1 108.97,44.58 108.97,46.99 R3.1 109.09,46.99 v110.36,48.26 107.7,50.93 107.7,52.96 107.57,53.09 | 108.2,41.02 106.43,39.24 105.79,39.24 103.63,37.08 103.63,36.83 C1.2 103.38,36.7 103.12,36.45 101.98,36.45 98.04,32.51 98.04,30.23 | 44.07,14.61 46.23,14.61 C29.2 | v51.44,8.51 52.83,8.51 53.98,7.37 U$4.P55 | 113.28,3.56 113.28,7.87 112.39,8.76 109.47,8.76 R29.1 109.22,8.76 106.17,11.81 | 113.28,3.56 113.28,2.29 112.9,1.91 111.25,1.91 110.24,2.92 110.24,3.17 C2.2 | 113.28,3.56 121.28,3.56 123.83,6.1 123.83,8.13 J7.3 | 36.2,35.31 39.05,32.45 | 39.05,32.45 40.51,30.99 41.53,30.99 C35.2 | 36.2,35.31 v35.31,34.42 | U3.29 47.62,33.4 v47.62,28.45 47.5,28.32 46.86,28.32 43.43,24.89 41.66,24.89 41.53,25.02 40.51,25.02 39.75,24.26 39.75,23.24 | C36.2 60.2,24.89 58.04,22.73 57.4,22.73 U2.4 | 57.15,15.88 54.23,18.8 54.23,19.81 57.02,22.61 U2.4 | 39.75,23.24 42.93,20.07 43.31,20.07 44.07,19.3 44.07,14.61 | 39.75,23.24 v39.12,22.61 | 106.17,11.81 102.87,11.81 101.47,10.41 101.47,10.03 98.93,7.49 J5.P$1 98.81,5.84 93.34,5.84 91.82,4.32 88.65,4.32 86.49,6.48 | 82.8,15.75 79.5,12.45 U$4.P73 | 82.8,15.75 84.2,17.14 84.2,18.29 84.07,18.41 84.07,20.7 83.06,21.72 82.8,21.72 C26.2 | 107.57,26.67 107.57,15.88 106.3,14.61 106.3,11.94 106.17,11.81 | 98.04,30.23 98.04,28.96 96.14,27.05 95.89,27.05 C17.2 95.76,27.18 93.98,27.18 88.9,32.26 v88.9,32.64 | 98.04,30.23 v97.41,30.23 | v84.07,14.48 82.8,15.75 | 86.49,6.48 v86.49,12.06 | 57.15,15.88 57.28,16 61.59,16 65.41,12.19 66.93,12.19 C21.2 67.18,12.19 68.33,12.19 72.9,16.76 72.9,17.78 72.26,18.41 72.26,19.81 C11.2
  Bottom 0.508: 73.91,35.69 v73.03,34.8 | 21.46,1.14 9.78,1.14 7.87,3.05 C14.2 | 21.46,1.14 78.87,1.14 84.07,6.35 86.36,6.35 86.49,6.48 | v18.54,15.37 18.54,14.22 21.46,11.3 21.46,4.06 | 21.46,1.14 21.46,4.06 | v39.12,32.51 39.05,32.45 | v80.77,65.53 81.41,65.53 88.9,58.04 88.9,47.12 87.25,45.47 79.5,45.47 U$4.P99 | 111.89,29.84 108.33,33.4 108.33,40.89 108.2,41.02 | 107.57,53.09 98.93,53.09 T1.2 | 107.57,53.09 109.09,54.61 D1.A | v114.55,69.85 113.16,68.45 J6.8 | 119,65.02 119,58.55 118.49,58.04 118.49,56.52 | 119,65.02 v119,67.44 | J8.3 118.49,56.52 | v108.2,51.56 108.2,52.07 112.52,56.39 118.36,56.39 118.49,56.52 | 14.35,34.67 12.57,32.89 U8.1 | 14.35,34.67 16.13,36.45 18.03,36.45 18.41,36.07 18.41,34.42 17.4,33.4 17.14,33.4 C19.2 | v120.02,65.02 119,65.02 | C18.2 16.51,25.4 17.4,24.51 17.4,22.86 16.51,21.97 14.73,21.97 12.83,20.07 12.83,19.05 13.59,18.29 v15.11,18.29
  pour Top (isolate 0.813, rank 6): 0,78.74 0,-0.64 128.27,-0.64 128.27,78.74
  pour Bottom (isolate 0.813, rank 6): 0,78.74 0,41.27 22.23,41.27 22.23,0 127.64,0 127.64,11.43 111.76,11.43 111.76,41.27 127.64,41.27 127.64,78.74
JOY1  (via drill 0.51)
  Top 0.406: v59.44,71.12 55.37,71.12 v48.9,64.64 | v37.47,62.23 35.31,62.23 33.78,60.71 U$4.P141
  Bottom 0.406: J6.1 104.65,65.91 99.44,71.12 v59.44,71.12 | v48.9,64.64 46.23,64.64 43.94,66.93 41.02,66.93 39.62,65.53 39.62,62.99 38.86,62.23 v37.47,62.23
JOY2  (via drill 0.51)
  Top 0.406: v58.29,68.33 56.64,68.33 v50.93,62.61
  Bottom 0.406: J6.2 108.33,65.91 106.68,64.26 88.77,64.26 82.55,70.48 60.45,70.48 v58.29,68.33 | v50.93,62.61 49.02,60.71 U$4.P129
JOY3  (via drill 0.51)
  Top 0.406: v110.36,64.52 99.31,64.52 99.06,64.77 86.61,64.77 v82.04,69.34 | v72.64,64.26 77.09,64.26 80.14,61.21 80.14,60.2 76.96,57.02 76.2,57.02 74.17,54.99 70.36,54.99 v69.22,53.85 | v67.69,56.39 66.55,56.39 64.14,53.98 64.14,53.85 63.5,53.21 56.39,53.21 51.56,58.04 U$4.P128
  Bottom 0.406: v110.36,64.52 J6.3 | v82.04,69.34 77.72,69.34 v72.64,64.26 | v69.22,53.85 66.29,53.85 65.66,54.48 65.66,55.5 66.55,56.39 v67.69,56.39
JOY4  (via drill 0.51)
  Top 0.406: v112.9,64.39 111.89,64.39 110.87,63.37 99.57,63.37 98.81,64.14 85.6,64.14 78.99,70.74 v78.99,72.26 | v38.99,74.55 30.99,66.55 v30.23,66.55 | v36.7,56.01 52.7,56.01 56.64,52.07 v57.66,52.07
  Bottom 0.406: v112.9,64.39 114.43,65.91 J6.4 | v78.99,72.26 76.71,74.55 v38.99,74.55 | v30.23,66.55 30.23,61.85 29.72,61.34 29.72,57.53 31.24,56.01 v36.7,56.01 | v57.66,52.07 57.66,54.1 61.59,58.04 U$4.P120
JOY5  (via drill 0.51)
  Top 0.406: v36.83,53.72 39.12,53.72 v40.26,54.86
  Bottom 0.406: J6.6 103,68.45 95.76,75.69 32.64,75.69 24.51,67.56 24.51,61.72 31.24,54.99 31.24,54.36 31.88,53.72 v36.83,53.72 | v40.26,54.86 40.26,57.02 41.27,58.04 U$4.P136
JOY6  (via drill 0.51)
  Top 0.406: v94.87,59.44 90.17,59.44 88.39,57.66 v82.93,57.66 | v77.85,59.56 74.93,56.64 v73.03,56.64
  Bottom 0.406: J6.5 116.46,65.91 113.79,63.25 98.68,63.25 v94.87,59.44 | v82.93,57.66 79.76,57.66 v77.85,59.56 | v73.03,56.64 70.74,56.64 69.34,58.04 U$4.P114
JOY7  (via drill 0.51)
  Top 0.406: v114.94,71.5 81.41,71.5 79.5,73.41 v76.2,73.41 | v59.44,73.41 59.44,72.77 61.59,70.61 61.59,60.71 U$4.P119
  Bottom 0.406: v114.94,71.5 115.82,70.61 115.82,68.45 J6.9 | v59.44,73.41 v76.2,73.41
L-OUT  (via drill 0.51)
  Top 0.406: v12.7,67.44 15.49,70.23 v15.49,74.8 17.14,76.45 v21.72,76.45 | v115.7,47.12 115.7,50.16 115.95,50.42 115.95,60.07 115.82,60.2 115.82,62.48 120.14,66.8 120.14,67.94 111.25,76.83 v72.77,76.83
  Bottom 0.406: R22.2 C3.1 15.49,76.71 v15.49,74.8 | v12.7,67.44 11.81,67.44 9.53,65.15 J4.P$2 | J8.12 122.05,44.83 120.65,43.43 119.38,43.43 v115.7,47.12 | v72.77,76.83 22.1,76.83 v21.72,76.45
LED  (via drill 0.51)
  Top 0.406: R6.1 98.93,49.91 v98.81,49.78 | v78.99,67.31 69.34,76.96 24.77,76.96 16,68.2 16,50.29 22.99,43.31 v22.99,42.04 | v26.42,37.97 27.18,37.97 29.59,35.56 40.51,35.56 41.91,34.16 70.74,34.16 76.83,40.26 U$4.P96
  Bottom 0.406: v98.81,49.78 98.81,50.04 81.53,67.31 v78.99,67.31 | v22.99,42.04 26.42,38.61 v26.42,37.97
LEFT  (via drill 0.51)
  Top 0.406: v19.94,69.6 19.94,62.48 19.05,61.59 19.05,55.75 16.64,53.34 16.64,50.8 18.03,49.4 27.18,49.4 28.57,48.01 U$4.P7
  Bottom 0.406: v19.94,69.6 19.94,76.83 R22.1
N$1
  Bottom 0.406: C8.2 99.44,24.13 99.44,30.73 100.84,32.13 102.87,32.13 103.25,31.75 U4.6
N$2
  Bottom 0.406: C7.2 99.31,20.32 99.31,20.57 97.03,22.86 96.65,22.86 96.39,23.11 96.39,25.4 98.81,27.81 98.81,30.99 100.58,32.77 103,32.77 103.25,33.02 U4.7
N$3  (via drill 0.51)
  Top 0.406: v96.14,18.03 96.14,19.05 101.98,24.89 101.98,26.92 100.08,28.83 100.08,32.77 v101.22,33.91
  Bottom 0.406: v96.14,18.03 98.04,18.03 99.31,16.76 99.31,16.51 C6.2 | v101.22,33.91 102.87,33.91 103.25,34.29 U4.8
N$4  (via drill 0.51)
  Top 0.406: R32.2 95.25,28.07 97.54,25.78 97.79,25.78 R33.1 97.92,25.65 98.17,25.4 v100.84,25.4
  Bottom 0.406: v100.84,25.4 U4.1
N$5
  Top 0.406: LED1.A R6.2
N$6  (via drill 0.51)
  Top 0.406: Y1.2 106.3,20.32 108.46,18.16 112.52,18.16 114.3,19.94 114.3,20.95 113.67,21.59 112.52,21.59 111.25,22.86 111.25,32.13 v107.06,36.32
  Bottom 0.406: U4.3 104.14,27.94 105.66,29.46 105.66,34.67 105.54,34.8 105.54,36.83 C1.1 105.66,36.32 v107.06,36.32
N$7  (via drill 0.51)
  Top 0.406: v114.55,32.26 114.55,26.29 113.28,25.02 113.28,22.86 114.94,21.21 114.94,19.68 112.78,17.53 97.54,17.53 90.81,10.79 90.81,9.65 v85.22,4.06 | v81.92,0.76 4.06,0.76 0.64,4.19 0.64,18.54 4.06,21.97 4.06,36.45 2.67,37.85 2.67,39.5 1.27,40.89 1.27,41.91 v2.54,43.18
  Bottom 0.406: U4.10 113.79,33.02 v114.55,32.26 | v81.92,0.76 v85.22,4.06 | C13.+ v2.54,43.18
N$8
  Top 0.406: LED2.A 17.14,10.67 15.75,10.67 13.72,12.7 R7.2
N$9
  Bottom 0.406: C13.- 5.84,48.26 10.03,52.45 10.03,54.48 9.27,55.24 9.27,57.15 R4.2
N$10
  Bottom 0.406: U$3.2 7.62,60.83 7.37,60.58 7.37,57.15 R4.1 7.49,57.02 7.62,56.9 7.62,53.47 U$3.2@1
N$11
  Bottom 0.406: T1.1 98.93,54.86 100.97,54.86 101.22,54.61 R28.1
N$12  (via drill 0.51)
  Top 0.406: v117.73,62.23 119.25,62.23 120.78,63.75 121.79,63.75 125.35,60.2 v125.35,38.73 | v125.35,35.43 125.6,35.43 126.75,34.29 126.75,24.13 v126.24,23.62 | v111.89,7.49 116.46,12.06 117.22,12.06 117.35,12.19 122.56,12.19 v126.62,16.26
  Bottom 0.406: D1.C R28.2 103.12,54.74 103.12,56.77 108.58,62.23 v117.73,62.23 | C2.1 112.01,3.17 112.01,5.21 111.51,5.71 C5.1 111.89,5.59 v111.89,7.49 | v125.35,38.73 126.49,37.59 126.49,36.58 v125.35,35.43 | v126.62,16.26 126.62,23.24 v126.24,23.62
N$13
  Bottom 0.406: R11.1 107.31,4.83 108.58,4.83 109.47,5.71 C5.2
N$14
  Bottom 0.406: R11.2 107.31,2.92 107.06,2.92 106.05,3.94 106.05,5.59 107.57,7.11 107.57,8.26 R29.2 107.44,8.38 105.03,8.38 104.01,9.4 J5.P$2
N$15
  Top 0.406: R24.2 25.4,59.44 25.4,58.8 28.57,55.63 U$4.P1
N$16
  Bottom 0.406: R10.1 76.2,4.95 76.2,8 74.42,9.78 U$4.P72
N$17
  Bottom 0.406: R23.1 33.91,12.95 33.91,10.03 33.78,9.91 U$4.P40
N$18
  Bottom 0.406: R8.1 121.67,8.38 121.79,8.26 J7.1
N$19
  Bottom 0.406: R9.1 126.87,9.65 124.97,9.65 123.95,10.67 J7.5
N$20
  Bottom 0.406: R5.1 110.36,68.45 J6.7
N$21
  Bottom 0.508: L2.1 11.05,5.71 11.05,7.37 10.16,8.26 U6.2 U6.4
  pour Bottom (isolate 0.813, rank 6): 0.64,19.68 0.64,5.08 17.14,5.08 17.14,19.68
N$22
  Bottom 0.508: L5.1 120.65,31.75 121.28,31.11 U7.2 U7.4
  pour Bottom (isolate 0.813, rank 6): 115.57,34.92 115.57,13.34 127.64,13.34 127.64,34.92
N$23
  Bottom 0.508: L3.1 U8.2 U8.4
  pour Bottom (isolate 0.813, rank 6): 1.91,38.1 1.91,23.5 15.88,23.5 15.88,38.73 1.91,38.73
N$24  (via drill 0.51)
  Top 0.406: v101.22,29.34 101.6,28.96 106.05,28.96 L4.2
  Bottom 0.406: v101.22,29.34 103.12,29.34 103.25,29.21 U4.4
N$25
  Top 0.305: 4.7,9.65 J1.1
  Top 0.508: 4.7,9.65 5.46,9.65 6.22,8.89 7.37,8.89 L1.P$1
N$26
  Top 0.305: 4.7,6.86 J1.5
  Top 0.508: 4.7,6.86 5.46,6.86 6.22,7.62 7.37,7.62 L1.P$2
PS2_CLK  (via drill 0.51)
  Top 0.406: v121.67,15.37 121.67,29.46 125.35,33.15 v125.35,33.78 | v115.7,40.39 115.7,40.77 107.82,48.64 98.3,48.64 95,51.94 95,57.15 94.36,57.78 89.41,57.78 87.25,55.63 79.5,55.63 U$4.P107
  Bottom 0.406: 126.75,11.81 R9.2 126.62,11.81 125.22,11.81 v121.67,15.37 | v125.35,33.78 127.13,35.56 127.13,38.61 124.84,40.89 116.2,40.89 v115.7,40.39
PS2_DATA  (via drill 0.51)
  Top 0.406: v116.97,14.35 113.67,14.35 113.03,13.72 97.54,13.72 v97.16,13.34 | v83.95,29.72 83.95,32.26 80.9,35.31 80.9,38.86 79.5,40.26 U$4.P95
  Bottom 0.406: v116.97,14.35 118.75,12.57 121.67,12.57 R8.2 | v97.16,13.34 91.44,13.34 88.14,16.64 88.14,22.1 88.52,22.48 88.52,25.15 v83.95,29.72
R  (via drill 0.51)
  Top 0.406: v107.57,12.57 v101.85,12.57 | v114.43,24.51 114.43,25.27 115.7,26.54 v115.7,33.91 | v103.76,38.99 v110.62,38.99 | v116.97,60.71 v121.41,60.71 | v104.27,56.26 104.27,52.32 v104.78,51.82
  Bottom 0.406: R3.2 106.68,46.99 105.92,47.75 104.9,47.75 | 104.9,47.75 104.65,47.75 104.01,47.12 R14.2 103.89,46.86 103.89,44.45 R17.2 103.89,44.32 103.89,42.04 R20.2 103.76,41.91 v103.76,38.99 | v101.85,12.57 101.85,19.94 100.2,21.59 99.82,21.59 97.54,23.88 97.54,24.13 C8.1 | v107.57,12.57 107.57,13.21 114.43,20.07 v114.43,24.51 | v110.62,38.99 v115.7,33.91 | J8.4 122.56,55.5 123.95,56.9 123.95,58.17 v121.41,60.71 | v116.97,60.71 108.71,60.71 v104.27,56.26 | v104.78,51.82 104.78,51.31 104.9,51.18 104.9,47.75
R0  (via drill 0.51)
  Top 0.406: v90.55,32.38 90.55,27.05 v86.74,23.24 | v74.93,14.86 74.93,15.62 72.52,18.03 v72.52,21.59
  Bottom 0.406: R20.1 100.97,41.91 98.55,39.5 97.66,39.5 v90.55,32.38 | v86.74,23.24 86.74,15.49 84.58,13.34 82.42,13.34 80.01,10.92 76.33,10.92 74.93,12.32 v74.93,14.86 | v72.52,21.59 75.95,21.59 76.83,22.48 U$4.P82
R1  (via drill 0.51)
  Top 0.406: v98.81,38.35 v98.81,41.4 | v95,31.75 94.74,31.75 93.47,30.48 93.47,16.51 82.68,5.71 v81.66,5.71 | v28.57,14.86 v24,10.29 | v36.83,23.88 40.89,23.88 v41.02,23.75 | v54.48,29.59 55.63,30.73 67.56,30.73 70.87,27.43 71.88,27.43 73.03,28.57 v73.03,28.96
  Bottom 0.406: v98.81,41.4 101.85,44.45 R17.1 | v98.81,38.35 98.81,35.56 v95,31.75 | v81.66,5.71 80.9,5.71 77.22,2.03 30.61,2.03 24,8.64 v24,10.29 | v28.57,14.86 28.57,15.62 v36.83,23.88 | v41.02,23.75 43.69,23.75 47.24,27.3 48.13,27.3 50.42,29.59 v54.48,29.59 | v73.03,28.96 73.53,28.96 77.34,25.15 79.38,25.15 U$4.P83
R2  (via drill 0.51)
  Top 0.406: v90.17,37.97 v90.17,42.93
  Bottom 0.406: R14.1 94.23,46.99 v90.17,42.93 | v90.17,37.97 88.77,37.97 83.44,32.64 83.44,32 79.5,28.07 79.5,27.69 U$4.P85
R-OUT  (via drill 0.51)
  Top 0.406: v117.73,43.31 117.73,42.67 v120.65,39.75 | v125.35,37.08 127.38,35.05 127.38,19.3 121.28,13.21 115.82,13.21 105.41,2.79 100.58,2.79 98.93,1.14 83.19,1.14 82.42,1.91 20.57,1.91 20.32,1.65 7.11,1.65 2.79,5.97 2.79,10.79 6.22,14.22 6.22,20.57 7.11,21.46 8.64,21.46 10.67,23.5 10.67,38.23 14.73,42.29 14.73,66.29 v14.22,66.8
  Bottom 0.406: J4.P$3 9.53,75.06 11.56,73.03 R21.2 13.72,73.03 13.72,72.77 14.86,71.63 14.86,69.22 C4.1 14.73,69.09 14.22,68.58 v14.22,66.8 | 122.68,48.01 J8.10 122.68,47.24 122.68,46.74 123.95,45.47 123.95,44.2 122.56,42.8 118.24,42.8 v117.73,43.31 | v120.65,39.75 122.68,39.75 v125.35,37.08
RIGHT
  Bottom 0.406: R21.1 15.62,73.03 15.62,72.26 20.83,67.06 23.11,67.06 23.88,66.29 23.88,52.2 23.37,51.69 23.37,50.67 26.04,48.01 U$4.P8
SD_CS  (via drill 0.51)
  Top 0.406: v22.1,28.32 18.41,32 17.14,32 J2.2 | v34.8,26.42 36.32,26.42 42.04,32.13 43.56,32.13 44.07,32.64 72.01,32.64 v72.52,33.15 | v75.06,23.62 75.06,19.3 79.38,14.99 U$4.P75
  Bottom 0.406: v22.1,28.32 22.86,28.32 24.77,26.42 v34.8,26.42 | v72.52,33.15 72.52,31.37 70.23,29.08 70.23,28.07 74.68,23.62 v75.06,23.62
SD_MISO  (via drill 0.51)
  Top 0.406: v18.67,18.41 18.67,25.53 17.65,26.54 17.14,26.54 J2.7 | v71.37,28.57 70.61,28.57 67.82,31.37 44.58,31.37 v38.23,25.02 | v30.1,18.8 v33.4,18.8
  Bottom 0.406: 16.64,16.64 18.41,18.41 v18.67,18.41 | 16.64,16.64 13.34,13.34 13.34,11.56 14.35,10.54 14.61,10.54 R34.1 | v71.37,28.57 72.14,27.81 73.66,27.81 78.87,22.61 79.38,22.61 U$4.P81 | v38.23,25.02 38.23,23.62 v33.4,18.8 | v30.1,18.8 27.56,18.8 25.27,16.51 16.76,16.51 16.64,16.64
SD_MOSI  (via drill 0.51)
  Top 0.406: v14.1,19.56 11.3,22.35 11.3,25.78 16.38,30.86 17.02,30.86 J2.3 | v22.73,18.8 25.27,18.8 25.78,18.29 28.96,18.29 29.59,17.65 40.01,17.65 40.64,17.02 47.12,17.02 47.62,17.53 52.07,17.53 54.99,14.61 56.26,14.61 56.77,15.11 59.05,15.11 62.87,11.3 68.45,11.3 v68.71,11.05
  Bottom 0.406: v14.1,19.56 15.75,21.21 20.32,21.21 v22.73,18.8 | v68.71,11.05 69.22,11.05 74.17,16 75.82,16 76.83,14.99 U$4.P76
SD_SCK  (via drill 0.51)
  Top 0.406: v22.61,15.37 21.08,16.89 21.08,25.4 17.78,28.7 17.14,28.7 J2.5 | v26.92,15.37 27.43,15.37 28.07,16 38.35,16 v38.48,15.88 | v41.15,18.16 41.78,18.16 42.29,17.65 46.86,17.65 47.88,18.67 v56.13,18.67 | v67.69,13.72 70.23,11.18 v70.23,10.41 | v82.17,16.89 v82.17,11.43
  Bottom 0.406: v26.92,15.37 v22.61,15.37 | v38.48,15.88 38.86,15.88 v41.15,18.16 | v56.13,18.67 56.13,18.03 57.4,16.76 64.64,16.76 v67.69,13.72 | v70.23,10.41 72.77,10.41 73.66,11.3 75.06,11.3 76.07,10.29 81.03,10.29 v82.17,11.43 | v82.17,16.89 80.01,16.89 79.5,17.4 U$4.P77
TCK  (via drill 0.51)
  Top 0.406: v113.28,52.45 112.01,52.45 111.89,52.32 110.87,52.32 106.68,56.52 106.68,57.28 102.11,61.85 82.55,61.85 v82.3,61.59 | v77.47,61.21 74.42,58.17 U$4.P110
  Bottom 0.406: v113.28,52.45 J8.5 | v82.3,61.59 81.03,61.59 80.64,61.21 v77.47,61.21
TDI  (via drill 0.51)
  Top 0.406: v111.38,53.47 102.11,62.74 86.11,62.74 77.34,71.5 v77.34,72.26 | v54.86,72.26 45.59,62.99 41.78,62.99 38.86,65.91 35.43,65.91 31.62,62.1 30.48,62.1 29.72,61.34 29.72,59.56 31.11,58.17 U$4.P144
  Bottom 0.406: J8.9 117.98,47.37 115.57,49.78 114.3,49.78 111.38,52.7 v111.38,53.47 | v54.86,72.26 v77.34,72.26
TDO  (via drill 0.51)
  Top 0.406: v114.43,51.31 111,51.31 106.05,56.26 106.05,57.02 101.85,61.21 83.57,61.21 82.8,60.45 81.79,60.45 80.39,61.85 v80.39,62.61 | v76.33,62.61 74.42,60.71 U$4.P109
  Bottom 0.406: J8.7 116.33,49.91 114.94,51.31 v114.43,51.31 | v76.33,62.61 v80.39,62.61
TMS  (via drill 0.51)
  Top 0.406: v112.52,48.9 105.41,56.01 105.41,56.77 101.6,60.58 83.82,60.58 80.26,57.02 78.36,57.02 76.96,55.63 U$4.P108
  Bottom 0.406: J8.11 119.63,44.83 115.57,48.9 v112.52,48.9
WR
  Bottom 0.406: U3.24 53.85,33.53 53.85,34.42 45.09,43.18 41.78,43.18 41.27,42.67 38.99,42.67 28.7,52.96 U$4.P3
XA0  (via drill 0.51)
  Top 0.406: v57.78,49.53 61.34,49.53 v66.8,54.99 | v74.42,62.61 66.17,62.61 64.26,60.71 U$4.P117
  Bottom 0.406: v57.78,49.53 57.78,46.35 U3.12 | v66.8,54.99 73.28,54.99 75.82,57.53 75.82,61.21 v74.42,62.61
XA1
  Bottom 0.406: U3.11 56.52,46.35 56.52,55.5 59.05,58.04 U$4.P122
XA2  (via drill 0.51)
  Top 0.406: v55.12,49.53 52.96,49.53 49.91,52.58 36.32,52.58 34.8,54.1 v34.8,54.86 | v32.38,54.86 29.08,58.17 29.08,62.87 33.66,67.44 36.2,67.44 37.59,68.83 v37.59,69.98
  Bottom 0.406: v55.12,49.53 55.12,46.35 U3.10 | v32.38,54.86 v34.8,54.86 | v37.59,69.98 37.59,69.22 38.61,68.2 49.02,68.2 56.52,60.71 U$4.P123
XA3
  Bottom 0.406: U3.9 53.98,46.35 53.98,55.5 56.52,58.04 U$4.P124
XA4  (via drill 0.51)
  Top 0.406: v51.94,48.9 49.91,48.9 48.51,50.29 39.88,50.29 38.86,51.31 34.29,51.31 30.1,55.5 30.1,56.26 28.45,57.91 v28.45,65.02
  Bottom 0.406: v51.94,48.9 52.58,48.26 52.58,46.35 U3.8 | v28.45,65.02 28.45,67.31 31.62,70.48 35.43,70.48 38.35,67.56 47.62,67.56 53.98,61.21 53.98,60.71 U$4.P125
XA5
  Bottom 0.406: U3.7 51.31,46.35 51.31,47.88 50.8,48.39 50.8,54.86 53.98,58.04 U$4.P126
XA6
  Bottom 0.406: U3.6 50.04,46.35 50.04,57.02 49.02,58.04 U$4.P130
XA7  (via drill 0.51)
  Top 0.406: v48.77,48.39 40.01,48.39 30.48,38.86 v30.48,38.48 | v26.04,67.44 v22.1,63.5 | v41.78,70.23 41.78,69.47 45.09,66.17 v45.09,64.14
  Bottom 0.406: v48.77,48.39 48.77,46.35 U3.5 | v30.48,38.48 28.45,38.48 22.61,44.32 22.61,49.66 22.1,50.16 v22.1,63.5 | v26.04,67.44 26.54,67.44 31.5,72.39 39.62,72.39 v41.78,70.23 | v45.09,64.14 45.09,61.98 46.35,60.71 U$4.P131
XA8  (via drill 0.51)
  Top 0.406: v56.13,29.59 65.28,29.59 v68.33,26.54 | v71.63,17.27 71.63,16.51 75.69,12.45 76.83,12.45 U$4.P74
  Bottom 0.406: v56.13,29.59 54.99,30.73 52.2,30.73 50.16,32.77 50.16,33.4 U3.27 | v68.33,26.54 68.33,21.72 71.5,18.54 71.5,17.4 v71.63,17.27
XA9  (via drill 0.51)
  Top 0.406: v42.42,40.39 44.07,42.04 44.07,45.09 41.91,47.24 v41.66,47.24 | v41.66,51.44 39.62,51.44 39.12,51.94 36.07,51.94 33.66,54.36 33.66,58.04 U$4.P142
  Bottom 0.406: v42.42,40.39 45.34,40.39 51.31,34.42 51.31,33.53 U3.26 | v41.66,51.44 v41.66,47.24
XA10  (via drill 0.51)
  Top 0.406: v67.18,43.31 76.83,52.96 U$4.P106
  Bottom 0.406: v67.18,43.31 64.26,43.31 55.24,34.29 55.24,33.53 U3.23
XA11  (via drill 0.51)
  Top 0.406: v42.42,42.04 42.42,43.31 42.93,43.81 42.93,44.83 41.66,46.1 40.64,46.1 v40.01,46.74
  Bottom 0.406: v42.42,42.04 44.96,42.04 52.58,34.42 52.58,33.53 U3.25 | v40.01,46.74 37.97,48.77 37.97,56.39 36.32,58.04 U$4.P140
XA12
  Bottom 0.406: U3.4 47.5,46.35 47.5,57.02 46.48,58.04 U$4.P132
XA13  (via drill 0.51)
  Top 0.406: v39.12,34.16 34.8,29.84 27.69,29.84 v26.04,31.5 | v21.34,36.32 21.34,38.35 22.1,39.12 22.1,40.13 17.91,44.32 v17.91,46.74 | v17.91,51.18 19.18,51.18 23.5,55.5 26.04,55.5 U$4.P2
  Bottom 0.406: v39.12,34.16 41.4,36.45 46.74,36.45 48.77,34.42 48.77,33.53 U3.28 | v26.04,31.5 26.04,33.02 22.73,36.32 v21.34,36.32 | v17.91,51.18 v17.91,46.74
XA14
  Bottom 0.406: U3.3 46.23,46.35 46.23,55.75 43.94,58.04 U$4.P134
XA15  (via drill 0.51)
  Top 0.406: v42.42,38.1 v42.42,35.31
  Bottom 0.406: v42.42,35.31 44.07,35.31 44.96,34.42 44.96,33.53 U3.31 | v42.42,38.1 30.1,50.42 28.7,50.42 U$4.P5
XA16  (via drill 0.51)
  Top 0.406: v36.7,46.74 36.7,46.35 29.21,38.86 28.07,38.86 26.67,40.26 v26.67,42.42 | v22.73,65.79 25.53,68.58 26.54,68.58 29.72,65.41 30.73,65.41 33.91,68.58 v35.69,68.58 | v38.48,63.5 41.27,60.71 U$4.P135
  Bottom 0.406: v36.7,46.74 37.85,45.59 41.66,45.59 42.8,46.74 42.8,47.37 43.31,47.88 44.32,47.88 44.96,47.24 44.96,46.35 U3.2 | v26.67,42.42 26.67,45.34 23.24,48.77 23.24,49.91 22.73,50.42 22.73,62.48 23.24,62.99 23.24,65.28 v22.73,65.79 | v35.69,68.58 35.69,67.82 38.48,65.02 v38.48,63.5
XA17  (via drill 0.51)
  Top 0.406: v41.78,44.32 37.97,44.32 30.99,37.34 28.7,37.34 26.92,39.12 v24.26,39.12 | v19.94,40.64 19.94,41.4 15.37,45.97 15.37,69.22 v21.08,74.93 | v25.53,70.48 30.99,70.48 v32.13,69.34
  Bottom 0.406: v41.78,44.32 43.69,46.23 U3.1 | v24.26,39.12 21.46,39.12 v19.94,40.64 | v25.53,70.48 v21.08,74.93 | v32.13,69.34 33.27,69.34 37.34,65.28 37.34,63.75 36.32,62.74 36.32,60.71 U$4.P139
XA18  (via drill 0.51)
  Top 0.406: v20.45,31.62 19.94,31.62 18.8,32.77 18.8,40.89 v16.26,43.43 | v20.19,50.55 23.62,50.55 26.04,52.96 U$4.P4
  Bottom 0.406: v20.45,31.62 24.51,27.56 39.88,27.56 41.78,25.65 43.18,25.65 46.86,29.34 46.86,32.38 46.35,32.89 46.35,33.4 U3.30 | v16.26,43.43 20.19,47.37 v20.19,50.55
XD0  (via drill 0.51)
  Top 0.406: v62.99,54.36 66.67,58.04 U$4.P116
  Bottom 0.406: v62.99,54.36 59.05,50.42 59.05,46.35 U3.13
XD1  (via drill 0.51)
  Top 0.406: v60.2,48.39 53.09,48.39 43.94,39.24 34.54,39.24 v32.13,36.83 | v21.08,65.91 21.08,67.69 29.08,75.69 58.8,75.69 64.01,70.48 v64.01,66.17
  Bottom 0.406: v60.2,48.39 60.2,46.35 U3.14 | v32.13,36.83 23.11,36.83 21.46,38.48 19.56,38.48 12.45,45.59 12.45,58.29 20.07,65.91 v21.08,65.91 | v64.01,66.17 66.67,66.17 67.06,66.55 68.07,66.55 69.22,65.41 69.22,60.71 U$4.P113
XD2  (via drill 0.51)
  Top 0.406: v62.99,49.28 71.75,58.04 U$4.P112
  Bottom 0.406: v62.99,49.28 61.59,47.88 61.59,46.35 U3.15
XD3  (via drill 0.51)
  Top 0.406: v70.23,18.16 70.23,17.02 76.33,10.92 80.01,10.92 80.9,11.81 80.9,30.73 v79.5,32.13 | v82.04,35.81 82.04,40.26 79.5,42.8 U$4.P97
  Bottom 0.406: v70.23,18.16 64.39,24 64.39,31.5 62.87,33.02 62.87,33.4 U3.17 | v79.5,32.13 79.5,33.27 v82.04,35.81
XD4  (via drill 0.51)
  Top 0.406: v64.9,37.59 71.63,37.59 76.83,42.8 U$4.P98
  Bottom 0.406: v64.9,37.59 61.59,34.29 61.59,33.53 U3.18
XD5  (via drill 0.51)
  Top 0.406: v39.62,18.8 v42.8,21.97 | v35.69,14.86 31.88,14.86 26.16,9.14 v25.15,9.14 | v85.09,26.8 85.09,34.67 v83.95,35.81 | v85.22,40.39 85.22,42.16 84.71,42.67 84.71,45.21 79.5,50.42 U$4.P103
  Bottom 0.406: v42.8,21.97 45.09,24.26 45.97,24.26 49.66,27.94 56.13,27.94 60.2,32 60.2,33.4 U3.19 | v35.69,14.86 v39.62,18.8 | v25.15,9.14 31.62,2.67 76.96,2.67 85.34,11.05 85.34,13.21 87.5,15.37 87.5,22.35 87.88,22.73 87.88,24 v85.09,26.8 | v83.95,35.81 83.95,39.12 v85.22,40.39
XD6  (via drill 0.51)
  Top 0.406: v65.53,39.12 76.83,50.42 U$4.P104
  Bottom 0.406: v65.53,39.12 63.88,39.12 59.05,34.29 59.05,33.53 U3.20
XD7  (via drill 0.51)
  Top 0.406: v64.14,40.26 64.14,44.96 v73.03,53.85
  Bottom 0.406: v64.14,40.26 63.75,40.26 57.78,34.29 57.78,33.53 U3.21 | v73.03,53.85 76.2,57.02 80.01,57.02 80.9,56.13 80.9,54.48 79.5,53.09 U$4.P105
